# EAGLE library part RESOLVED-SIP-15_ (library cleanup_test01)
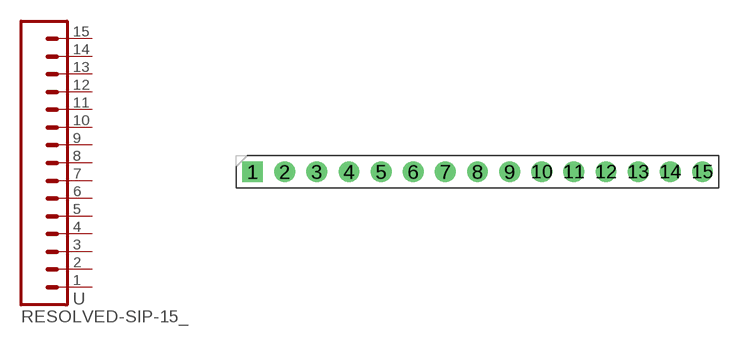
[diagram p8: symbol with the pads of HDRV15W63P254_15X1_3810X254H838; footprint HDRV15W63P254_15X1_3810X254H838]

Designator prefix -

## RESOLVED-SIP-15_2.54-SPACE-VERTICAL  [HDRV15W63P254_15X1_3810X254H838]
1  1  pas
2  2  pas
3  3  pas
4  4  pas
5  5  pas
6  6  pas
7  7  pas
8  8  pas
9  9  pas
10  10  pas
11  11  pas
12  12  pas
13  13  pas
14  14  pas
15  15  pas

## Footprint HDRV15W63P254_15X1_3810X254H838 (pad centres in mm)
drill 1.1 pad 1.65 square: 1 0,0
drill 1.1 pad 1.65: 2 2.54,0; 3 5.08,0; 4 7.62,0; 5 10.16,0; 6 12.7,0; 7 15.24,0; 8 17.78,0; 9 20.32,0; 10 22.86,0; 11 25.4,0; 12 27.94,0; 13 30.48,0; 14 33.02,0; 15 35.56,0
